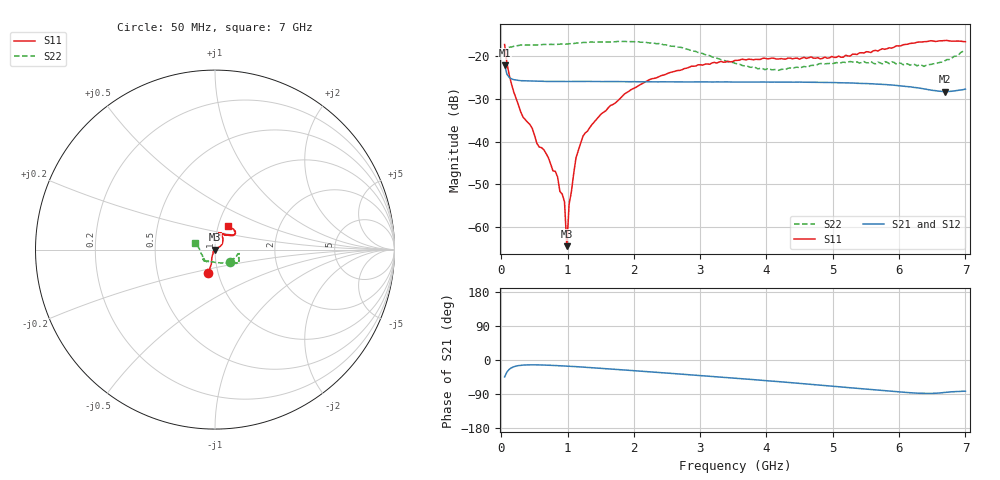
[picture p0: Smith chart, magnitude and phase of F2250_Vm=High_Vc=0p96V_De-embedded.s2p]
! Integrated Device Technology
! Corporate Headquarters
! 6024 Silver Creek Valley Road
! San Jose, CA 95138  USA
! Phone:  1-408-284-8200
! Toll Free:  1-800-223-1366
! Webpage:  http://www.idt.com/
! Timing and RF Division
! 515 Groton Road, Suite 102
! Westford, MA 01886-6024
! Device:  F2250
! Description: Voltage Variable RF Attenuator
! Frequency:  50.0 -  6000.00 MHz
! Package:  3x3 mm Thin QFN Plastic Package: 16 pin
! Ports:  2 RF, 3 DC
!  Pin  1  = GND
!  Pin  2  = NC
!  Pin  3  = RF1  = Port 1
!  Pin  4  = NC
!  Pin  5  = GND
!  Pin  6  = GND
!  Pin  7  = GND
!  Pin  8  = GND
!  Pin  9  = NC
!  Pin 10  = RF2  = Port 2
!  Pin 11  = NC
!  Pin 12  = GND
!  Pin 13  = GND
!  Pin 14  = VCNTRL
!  Pin 15  = VDD
!  Pin 16  = VMODE
! Vcntrl:  0.960 Volts
! Vmode:  +3.300 Volts
! Vdd:  +3.30  Volts
! Current:  1.321 mA
! Data:  The device was measured on a the F2250 evaluation board which has
!  individual transmission lines to the RF pins.  Data was collected
!  using a calibrated network analyzer.  The evaluation board was
!  de-embedded using a TRL calibration technique.
!  The reference plane is the edge of the package pin.
! Misc:  SN 10
!  Action Tracker AT0258
! Date Measured:  2014-11-26
! Date:  2015-10-15  MJV
! Note:
!  Integrated Device Technology supplies this data as a sample of measured
!  data at the package pin for this product.  Your particular data for this
!  product may vary.
!  Data was taken at 25 degrees C.
!  Integrated Device Technology reserves the right to change this data at anytime.
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# GHz S dB R 50
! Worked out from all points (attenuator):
!   201 points, 50 MHz to 7 GHz, reference 50 ohm
!   highest |S21| = -22.05 dB at 50 MHz (marker M1); lowest = -28.3 dB at 6.687 GHz (marker M2)
!   lowest |S11| = -64.5 dB at 988.2 MHz (marker M3), VSWR 1.00, Z = 50 - j0.0466 ohm
!   |S11| at or under -10 dB: start of sweep to end of sweep
!   |S22| runs from -23.3 to -16.5 dB; largest |S21 - S12| = 0.00021
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0.05  -17.21 -106.3  -22.05 -44.6  -22.07 -44.6  -19.44 -38.7
0.1195  -24.37 -107.8  -24.92 -24.7  -24.93 -24.7  -17.88 -13.0
0.29325  -33.00 -117.7  -25.68 -14.0  -25.67 -14.0  -17.34 -10.1
0.467  -36.85 -133.8  -25.78 -12.7  -25.76 -12.7  -17.38 -10.6
0.5365  -40.36 -138.8  -25.80 -12.8  -25.82 -12.8  -17.31 -11.9
0.64075  -41.85 -146.6  -25.85 -13.3  -25.84 -13.3  -17.20 -13.2
0.84925  -48.24 177.7  -25.85 -14.9  -25.86 -14.9  -17.18 -17.4
0.884  -51.63 170.1  -25.86 -15.2  -25.86 -15.2  -17.14 -18.3
0.9535  -54.07 -166.8  -25.87 -15.8  -25.88 -15.8  -17.16 -19.0
0.98825  -64.45 -51.0  -25.88 -16.1  -25.87 -16.1  -17.11 -19.5
1.023  -54.60 11.8  -25.88 -16.4  -25.87 -16.4  -17.03 -19.7
1.12725  -43.72 19.8  -25.87 -17.5  -25.86 -17.5  -16.89 -21.3
1.2315  -38.70 21.0  -25.85 -18.7  -25.85 -18.7  -16.74 -23.1
1.857  -28.82 32.8  -25.91 -26.4  -25.90 -26.4  -16.50 -28.9
2.37825  -24.73 42.5  -25.97 -32.9  -25.94 -33.0  -16.99 -33.1
3.525  -20.93 69.8  -26.01 -48.1  -26.00 -48.1  -21.62 -64.1
4.18525  -20.61 76.1  -26.02 -57.0  -26.03 -57.1  -23.28 -101.5
4.7065  -20.40 70.9  -26.07 -64.8  -26.07 -64.8  -22.09 -122.2
5.85325  -17.99 39.5  -26.66 -82.3  -26.64 -82.4  -21.70 -138.8
6.3745  -16.56 40.2  -27.60 -88.2  -27.60 -88.3  -22.35 -157.5
6.68725  -16.28 47.1  -28.25 -85.8  -28.23 -85.9  -21.05 175.2
7  -16.56 61.9  -27.67 -82.3  -27.67 -82.4  -18.60 160.7
